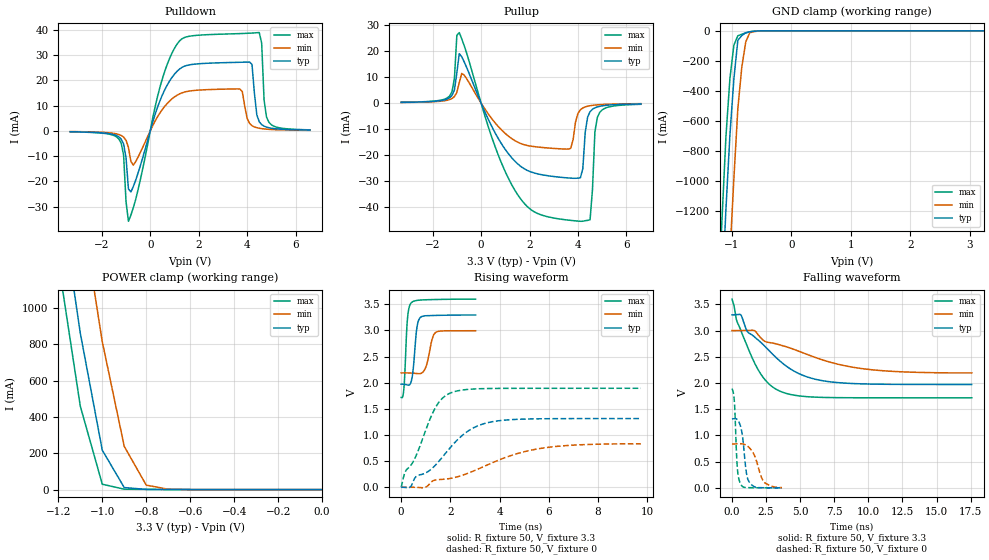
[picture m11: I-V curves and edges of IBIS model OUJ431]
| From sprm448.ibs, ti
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|CELL OPERATING IN NORMAL MODE WITHOUT PULLUP/PULLDOWN
|   Model Cell OUJ431
|OUJ431
[Model]   OUJ431
Model_type   3-state
Polarity   Non-Inverting
Enable   Active-Low
Cref =  15.0000pF
Rref =  100.0000M
Vref =  0V
Vmeas =  1.65
C_comp   2.2553p   1.8929p   2.9061p
[Temperature Range]   25   125   -40
[Voltage Range]   3.3   3   3.6
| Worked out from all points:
|   slope of the pulldown table from 0 to 0.495 V, typ, clamps not added: 35.1 ohm
|   slope of the pullup table from 0 to 0.495 V, typ, clamps not added: 49.5 ohm
|   GND clamp passes 1 mA (typ) near -0.56 V on its own axis
|   POWER clamp passes 1 mA (typ) near -0.78 V on its own axis
|   rising waveform, R_fixture 50, V_fixture 3.3: 20-80 % time 150ps typ, 222ps min, 117ps max; typ from 1.97 V to 3.29 V
|   rising waveform, R_fixture 50, V_fixture 0: 20-80 % time 1.7ns typ, 2.92ns min, 1.07ns max; typ from 0 V to 1.31 V
|   falling waveform, R_fixture 50, V_fixture 3.3: 20-80 % time 3.46ns typ, 5.64ns min, 2.01ns max; typ from 3.3 V to 1.97 V
|   falling waveform, R_fixture 50, V_fixture 0: 20-80 % time 341ps typ, 669ps min, 190ps max; typ from 1.31 V to 0.001 V
[POWER_clamp]
|   voltage   I(typ)   I(min)   I(max)
-3.3V     22.03A     22.67A     21.68A
-1.2V     1.688A     2.438A     1.256A
-1.167V   1.412A     2.154A     990.6mA
-1.133V   1.137A     1.87A      725mA
-1.1V     861.3mA    1.585A     459.4mA
-1.033V   431.8mA    1.071A     172.9mA
-1V       217.1mA    814.3mA    29.67mA
-900mV    11.25mA    237.8mA    2.263mA
-800mV    1.126mA    24.76mA    1.225mA
-700mV    476.2uA    1.927mA    593.6uA
-11.55fV  36.78pA    5.36nA     426.3fA
[Pulldown]
|   voltage   I(typ)   I(min)   I(max)
-3.3V     -336.6uA   -261.2uA   -375.2uA
-1.3V     -2.334mA   -1.416mA   -3.155mA
-1.1V     -5.177mA   -2.442mA   -9.521mA
-900mV    -22.98mA   -6.561mA   -35.8mA
-700mV    -22.04mA   -13.56mA   -30.48mA
1.1V      23.53mA    14.08mA    34.28mA
3.7V      27.17mA    16.59mA    38.53mA
4.1V      27.25mA    2.984mA    38.69mA
4.5V      3.644mA    1.04mA     38.94mA
4.7V      1.881mA    774.1uA    12.24mA
4.9V      1.25mA     615uA      3.388mA
6.6V      316.3uA    220.9uA    418.1uA
[Pullup]
|   voltage   I(typ)   I(min)   I(max)
-3.3V     267.2uA    225.9uA    296.8uA
-1.3V     2.024mA    1.343mA    2.701mA
-1.1V     5.048mA    2.506mA    9.537mA
-900mV    19.02mA    7.852mA    27.16mA
500mV     -10.09mA   -6.71mA    -14.73mA
1.5V      -23.34mA   -15.02mA   -35.16mA
3.7V      -28.94mA   -17.44mA   -45.22mA
4.1V      -28.81mA   -2.608mA   -45.57mA
4.5V      -3.335mA   -1.026mA   -44.98mA
4.7V      -1.842mA   -779.6uA   -11.04mA
4.9V      -1.259mA   -627.2uA   -3.6mA
6.6V      -333.1uA   -232.9uA   -483uA
[GND_clamp]
|   voltage   I(typ)   I(min)   I(max)
-3.3V     -22.43A    -23.21A    -22A
-1.233V   -2.349A    -3.221A    -1.841A
-1.167V   -1.762A    -2.627A    -1.261A
-1.1V     -1.19A     -2.042A    -704.7mA
-1.033V   -697.3mA   -1.495A    -319.5mA
-966.7mV  -321.8mA   -987mA     -95.62mA
-900mV    -63.49mA   -519.5mA   -33.01mA
-833.3mV  -31.57mA   -242.4mA   -22.69mA
-766.7mV  -12.54mA   -73.53mA   -13.85mA
-700mV    -6.383mA   -13.05mA   -6.471mA
-433.3mV  -65.52uA   -233.6uA   -21.24uA
3.233V    35.25pA    569.3nA    367.1fA
[Ramp]
| variable   typ   min   max
dV/dt_f  0.8030332/3.45176n   0.491836/5.711433n   1.137957/2.013579n
dV/dt_r  0.7955012/1.748024n   0.5078255/3.035144n   1.143394/1.089693n
R_load = 50
[Rising Waveform]
R_fixture = 50
V_fixture = 3.3
V_fixture_min = 3
V_fixture_max = 3.6
|   time   V(typ)   V(min)   V(max)
0s        1.972V     2.187V     1.718V
112ps     1.97V      2.188V     1.892V
264ps     1.956V     2.187V     3.257V
400ps     2.01V      2.185V     3.522V
496ps     2.288V     2.182V     3.557V
624ps     2.998V     2.176V     3.572V
776ps     3.246V     2.175V     3.581V
1ns       3.281V     2.295V     3.586V
1.4ns     3.287V     2.962V     3.591V
3.024ns   3.295V     2.994V     3.599V
[Rising Waveform]
R_fixture = 50
V_fixture = 0
V_fixture_min = 0
V_fixture_max = 0
|   time   V(typ)   V(min)   V(max)
0s        37.24pV    11.44nV    1.257pV
144ps     -838.8uV   168.5uV    273.2mV
368ps     2.905mV    313.4uV    405.5mV
592ps     198.2mV    -420.9uV   587.7mV
1.368ns   411.9mV    137mV      1.502V
1.992ns   756.7mV    169.1mV    1.801V
2.736ns   1.082V     272.2mV    1.873V
3.752ns   1.258V     478.7mV    1.89V
5.896ns   1.311V     759.4mV    1.893V
9.744ns   1.314V     831.4mV    1.893V
[Falling Waveform]
R_fixture = 50
V_fixture = 3.3
V_fixture_min = 3
V_fixture_max = 3.6
|   time   V(typ)   V(min)   V(max)
0s        3.3V       3V         3.6V
320ps     3.304V     3V         3.213V
680ps     3.29V      3.001V     2.982V
1.128ns   2.982V     3.003V     2.697V
1.76ns    2.854V     2.976V     2.329V
2.624ns   2.644V     2.778V     2.005V
3.592ns   2.402V     2.721V     1.837V
7.176ns   2.024V     2.399V     1.723V
11.1ns    1.976V     2.234V     1.718V
17.58ns   1.972V     2.193V     1.718V
[Falling Waveform]
R_fixture = 50
V_fixture = 0
V_fixture_min = 0
V_fixture_max = 0
|   time   V(typ)   V(min)   V(max)
0s        1.314V     837.5mV    1.893V
184ps     1.32V      838.2mV    1.609V
336ps     1.313V     840.4mV    632.2mV
416ps     1.296V     841.4mV    308.7mV
624ps     1.177V     842.4mV    80.57mV
792ps     945.7mV    838.2mV    21.77mV
1.064ns   276.4mV    810.3mV    6.275mV
1.296ns   100.2mV    758.9mV    4.346mV
2.328ns   3.157mV    119.4mV    1.422mV
3.664ns   1.441mV    6.132mV    485.1uV
